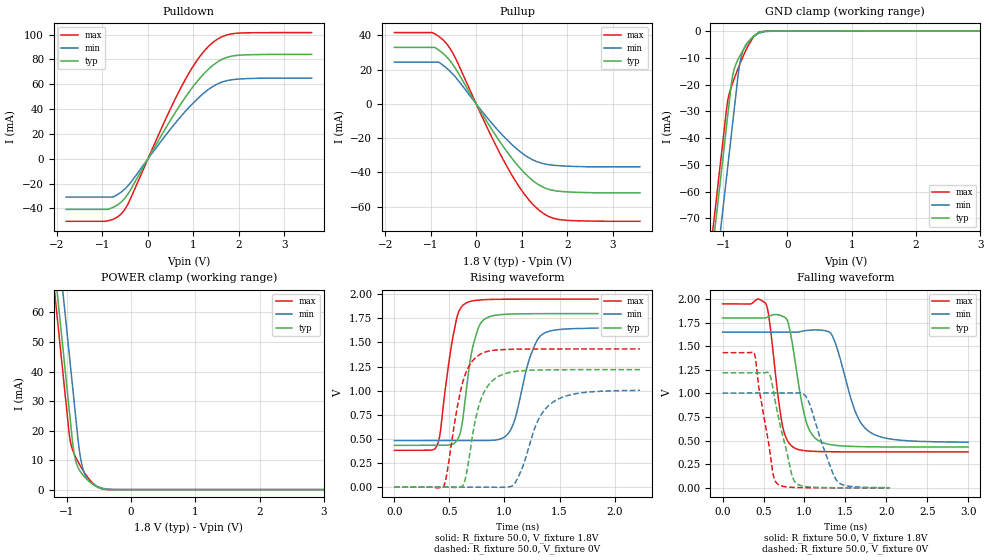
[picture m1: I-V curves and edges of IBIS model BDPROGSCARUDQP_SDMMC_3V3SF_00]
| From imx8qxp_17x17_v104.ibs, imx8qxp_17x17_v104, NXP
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[Model]   BDPROGSCARUDQP_SDMMC_3V3SF_00
Model_type I/O
Polarity   Non-Inverting
Enable   Active-Low
| CAP_THRESHOLD on pad IO is "CMOS" :
| Rising=10.0% of vdde1v8   Falling=90.0% of vdde1v8
| C_comp min and max val. don't necessarily correlate with the min and max pvt
| but are the smallest and greatest pad capacitance found.
| var   typ   min   max
C_comp   1.39830pF  1.34155pF  1.49815pF
Vinl = 580.0mV
Vinh = 1.27V
Vmeas = 900.0mV   | Reference voltage for timing measurements
Cref  = 15.0pF   | Timing specification test load capacitance value
Rref  = 1.0MOhm   | Timing specification test load resistance value
Vref  = 1.8V   | Timing specification test load voltage
[Model Spec]
| TIME_THRESHOLD on pin ZI is "CORE" :
| Rising=50.0% of vdd   Falling=50.0% of vdd
Vmeas 900.00000mV 825.00000mV 975.00000mV
Vref 1.80000V 1.65000V 1.95000V
| variable   typ   min   max
[Temperature Range] 25.0 125.0 -40.0
| variable   typ   min   max
[Voltage Range] 1.8V 1.65V 1.95V
| variable   typ   min   max
[POWER Clamp Reference] 1.8V 1.65V 1.95V
| variable   typ   min   max
[GND Clamp Reference] 0V 0V 0V
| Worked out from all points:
|   slope of the pulldown table from 0 to 0.27 V, typ, clamps not added: 15.6 ohm
|   slope of the pullup table from 0 to 0.27 V, typ, clamps not added: 22.9 ohm
|   GND clamp passes 1 mA (typ) near -0.48 V on its own axis
|   POWER clamp passes 1 mA (typ) near -0.53 V on its own axis
|   rising waveform, R_fixture 50.0, V_fixture 1.8V: 20-80 % time 107ps typ, 157ps min, 115ps max; typ from 0.433 V to 1.8 V
|   falling waveform, R_fixture 50.0, V_fixture 1.8V: 20-80 % time 167ps typ, 251ps min, 132ps max; typ from 1.8 V to 0.433 V
|   rising waveform, R_fixture 50.0, V_fixture 0V: 20-80 % time 139ps typ, 204ps min, 139ps max; typ from 0 V to 1.22 V
|   falling waveform, R_fixture 50.0, V_fixture 0V: 20-80 % time 187ps typ, 230ps min, 162ps max; typ from 1.22 V to 0 V
[POWER Clamp]
-1.8V     205.4mA    224.3mA    197mA
-1.18V    73.7mA     92.59mA    65.32mA
-1.15V    67.33mA    86.21mA    58.94mA
-1.12V    60.95mA    79.84mA    52.57mA
-1.06V    48.21mA    67.09mA    39.82mA
-1.04V    43.96mA    62.84mA    35.57mA
-950mV    24.83mA    43.72mA    17.27mA
-870mV    10.67mA    26.72mA    11.43mA
-810mV    6.903mA    14.47mA    8.897mA
-750mV    5.031mA    7.231mA    6.647mA
-550mV    1.187mA    1.353mA    1.363mA
3.6V      0A         0A         0A
[GND Clamp]
-1.8V     -216.7mA   -235.8mA   -210.3mA
-1.21V    -91.31mA   -110.4mA   -84.92mA
-1.12V    -72.19mA   -91.31mA   -65.8mA
-1.04V    -55.19mA   -74.31mA   -48.8mA
-940mV    -33.94mA   -53.06mA   -27.67mA
-860mV    -17.66mA   -36.06mA   -19.86mA
-820mV    -13.54mA   -27.56mA   -17.22mA
-770mV    -10.64mA   -16.96mA   -14.08mA
-730mV    -8.79mA    -10.76mA   -11.68mA
-640mV    -5.176mA   -4.882mA   -6.772mA
-450mV    -492.8uA   -817.4uA   -452.4uA
3.6V      109.1uA    87.23uA    140.4uA
| variable   typ   min   max
[Pullup Reference] 1.8V 1.65V 1.95V
| variable   typ   min   max
[Pulldown Reference] 0V 0V 0V
[Pullup]
-1.8V     33.01mA    24.43mA    41.69mA
-970mV    33.01mA    24.43mA    41.69mA
-830mV    31.61mA    24.43mA    39.61mA
-650mV    27.45mA    20.88mA    35.09mA
-450mV    20.46mA    15.52mA    26.43mA
230mV     -10.11mA   -7.67mA    -13.19mA
650mV     -26.95mA   -20.22mA   -35.31mA
1.07V     -40.53mA   -29.91mA   -53.1mA
1.41V     -47.79mA   -34.4mA    -62.68mA
1.65V     -50.28mA   -35.67mA   -66.34mA
1.92V     -51.25mA   -36.24mA   -67.83mA
3.6V      -51.91mA   -36.69mA   -68.55mA
[Pulldown]
-1.8V     -40.72mA   -30.81mA   -50.32mA
-880mV    -40.72mA   -30.81mA   -49.95mA
-770mV    -39.14mA   -30.78mA   -48.76mA
-550mV    -33.42mA   -25.62mA   -42.78mA
-410mV    -26.53mA   -20.44mA   -34.14mA
310mV     19.77mA    15.24mA    25.67mA
740mV     45.16mA    34.78mA    58.35mA
1.07V     61.77mA    47.68mA    78.8mA
1.41V     74.77mA    57.84mA    93.2mA
1.65V     80.47mA    62.07mA    98.65mA
1.92V     83.13mA    63.99mA    101mA
3.6V      84.07mA    64.91mA    101.7mA
[Ramp]
dV/dt_r 730.88031mV/139.16999ps 602.53977mV/204.04864ps 857.11439mV/139.26821ps
dV/dt_f 819.81631mV/166.75087ps 700.29607mV/250.61073ps 940.88152mV/131.63143ps
R_load = 50.0
| Removed startup time: 0s 0s 0s  .
| Removed end time: 1.83ns.
[Rising Waveform]
R_fixture   = 50.0
V_fixture   = 1.8V
V_fixture_min = 1.65V
V_fixture_max = 1.95V
0s        432.9mV    482.2mV    381mV
380ps     433mV      482.2mV    414.4mV
530ps     444.8mV    482.2mV    1.547V
630ps     778.7mV    482.2mV    1.892V
710ps     1.442V     482.2mV    1.931V
820ps     1.742V     482.4mV    1.944V
1.06ns    1.794V     602.6mV    1.948V
1.22ns    1.798V     1.305V     1.949V
1.33ns    1.799V     1.572V     1.949V
1.85ns    1.799V     1.649V     1.949V
| Removed startup time: 0s 0s 0s  .
| Removed end time: 2.98ns.
[Falling Waveform]
R_fixture   = 50.0
V_fixture   = 1.8V
V_fixture_min = 1.65V
V_fixture_max = 1.95V
0s        1.799V     1.649V     1.949V
530ps     1.802V     1.649V     1.949V
730ps     1.819V     1.649V     666.8mV
870ps     1.434V     1.649V     427.1mV
1.02ns    705.3mV    1.666V     392.5mV
1.18ns    496mV      1.672V     384.8mV
1.34ns    454.8mV    1.612V     382.3mV
1.61ns    438.5mV    834.1mV    381.1mV
1.78ns    435.4mV    603.3mV    380.9mV
3ns       432.9mV    482.2mV    381mV
| Removed startup time: 0s 0s 0s  .
| Removed end time: 2.21ns.
[Rising Waveform]
R_fixture   = 50.0
V_fixture   = 0V
V_fixture_min = 0V
V_fixture_max = 0V
0s        115uV      108.4uV    131uV
450ps     -393.5uV   158.4uV    10.76mV
570ps     -3.214mV   89.69uV    818.4mV
630ps     29.5mV     128uV      1.122V
780ps     888.6mV    -292.4uV   1.377V
900ps     1.112V     -2.045mV   1.418V
1.09ns    1.198V     32.56mV    1.43V
1.31ns    1.214V     703.8mV    1.432V
1.46ns    1.217V     895mV      1.432V
2.23ns    1.218V     1.004V     1.432V
| Removed startup time: 0s 0s 0s  .
| Removed end time: 2.02ns.
[Falling Waveform]
R_fixture   = 50.0
V_fixture   = 0V
V_fixture_min = 0V
V_fixture_max = 0V
0s        1.218V     1.004V     1.432V
390ps     1.218V     1.004V     1.421V
570ps     1.208V     1.004V     433.5mV
620ps     1.028V     1.004V     134.3mV
670ps     800.4mV    1.004V     42.3mV
840ps     158.6mV    1.004V     5.985mV
910ps     42.06mV    1.006V     3.411mV
1.05ns    10.31mV    916.5mV    1.437mV
1.41ns    1.368mV    62.51mV    400.4uV
2.04ns    122.1uV    119.5uV    135.6uV
